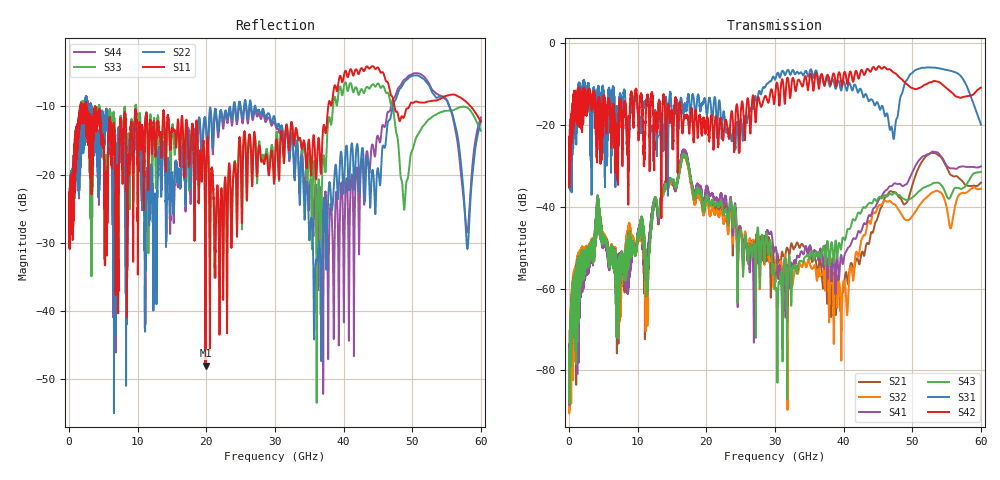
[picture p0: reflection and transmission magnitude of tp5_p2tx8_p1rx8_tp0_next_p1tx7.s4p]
! 100G CR Analysis
! File: tp5_p2tx8_p1rx8_tp0_next_p1tx7
! Description: 2m Cu Cable, OSFP, TP0-TP5
! Port Mapping
! Port1 -- P1RX8N
! Port2 -- P1TX7N
! Port3 -- P1RX8P
! Port4 -- P1TX7P
# GHz S MA R 50.00
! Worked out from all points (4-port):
!   6000 points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, 10 MHz to 60 GHz, reference 50 ohm
!   strongest paths, dB at 10 MHz, 15.01 GHz, 30.01 GHz, 45.01 GHz, 60 GHz:
!     S42: -27.9, -18.4, -12.9, -5.7, -10.8
!     S31: -27.9, -21.7, -8.9, -14.7, -19.9
!     S43: -80.2, -33.4, -59.0, -38.0, -31.4
!     S41: -78.7, -33.6, -50.1, -38.6, -30.1
!     S32: -84.4, -34.1, -56.4, -39.9, -35.6
!     S21: -81.7, -34.4, -58.1, -42.3, -34.1
!   lowest |S11| = -48.0 dB at 19.88 GHz (marker M1), VSWR 1.01, Z = 50 - j0.394 ohm
!   |S11| at or under -10 dB: start of sweep to 1.64 GHz; 3.811 GHz to 37.76 GHz (33.95 GHz wide, 163 % of centre); 47.4 GHz to 49.56 GHz (2.156 GHz wide, 4.45 % of centre)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
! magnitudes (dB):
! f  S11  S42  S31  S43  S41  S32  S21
! 10 MHz  -23.7  -27.9  -27.9  -80.2  -78.7  -84.4  -81.7
! 4.22 GHz  -11.2  -14.0  -10.6  -37.4  -37.3  -37.7  -37.6
! 19.88 GHz  -48.0  -21.9  -14.4  -38.6  -36.2  -39.5  -36.8
! 30.3 GHz  -15.3  -9.6  -7.4  -66.4  -52.4  -53.1  -51.7
! 35.87 GHz  -17.9  -7.8  -6.8  -51.3  -50.8  -54.6  -52.7
! 39.67 GHz  -6.0  -10.0  -11.5  -49.9  -51.8  -77.4  -63.0
! 60 GHz  -12.3  -10.8  -19.9  -31.4  -30.1  -35.6  -34.1
